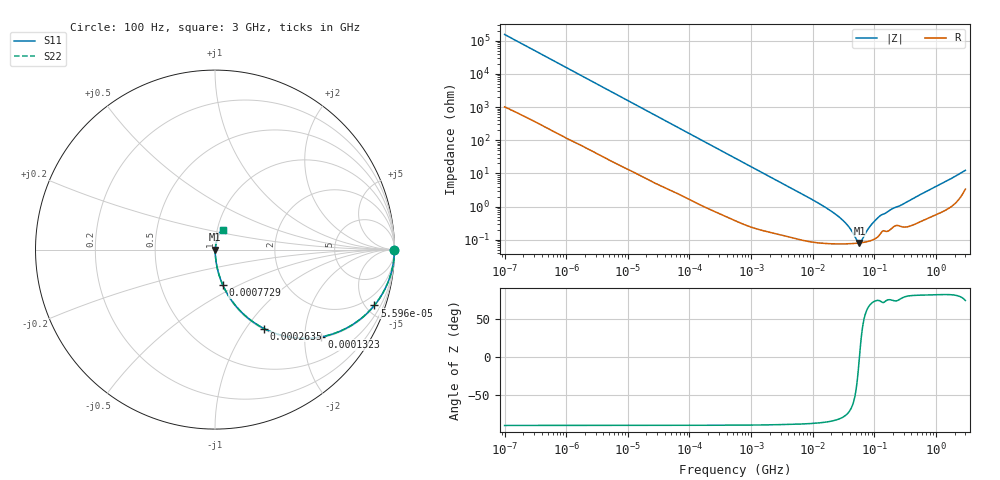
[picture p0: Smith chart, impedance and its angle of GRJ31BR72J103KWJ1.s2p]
!Murata Part Number: GRJ31BR72J103KWJ1
!These Parameters are Measured in Series Mode Connection
!Data Generated on Jun 19, 2026
!  o--ll--o
!Port1  Port2
!  o------o
!Operation Temp=25[degC], DC Bias Voltage=0[V]
!Freq. Start=100[Hz] Stop=3[GHz] 401[Steps]
# Hz S RI R 50
!Freq.(Hz) S11(Real) S11(Imag) S21(Real) S21(Imag) S12(Real) S12(Imag) S22(Real) S22(Imag)
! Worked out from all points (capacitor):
!   401 points, 100 Hz to 3 GHz, reference 50 ohm
!   read as one part in series: C = 10.3 nF near 109 Hz
!   lowest |Z| = 80.8 mohm at 57.2 MHz (marker M1)
!   series resonance near 57.24 MHz, so ESL is about 750 pH
!   S11 on the Smith chart (normalised r, x): 100 Hz: open; 55.95 kHz: 1.06, -5.68; 132.3 kHz: 1.03, -2.42; 263.5 kHz: 1.01, -1.22; 772.9 kHz: 1.01, -0.42; 3 GHz: 1.07, +0.24
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100  1 -0.00065  4.7e-06 0.00065  4.7e-06 0.00065  1 -0.00065
1788  0.9998 -0.0115  0.000221 0.0115  0.000221 0.0115  0.9998 -0.0115
10003  0.9954 -0.0632  0.00455 0.0632  0.00455 0.0632  0.9954 -0.0632
31977  0.9592 -0.1932  0.0408 0.1932  0.0408 0.1932  0.9592 -0.1932
55955  0.8874 -0.3113  0.1126 0.3113  0.1126 0.3113  0.8874 -0.3113
86054  0.7721 -0.4144  0.2279 0.4144  0.2279 0.4144  0.7721 -0.4144
132342  0.5924 -0.4862  0.4076 0.4862  0.4076 0.4862  0.5924 -0.4862
263501  0.273 -0.4398  0.727 0.4398  0.727 0.4398  0.273 -0.4398
547723  0.0828 -0.2692  0.9172 0.2692  0.9172 0.2692  0.0828 -0.2692
772864  0.0445 -0.1993  0.9555 0.1993  0.9555 0.1993  0.0445 -0.1993
2171352  0.00718 -0.0742  0.9928 0.0742  0.9928 0.0742  0.00718 -0.0742
9794414  0.00113 -0.0163  0.9989 0.0163  0.9989 0.0163  0.00113 -0.0163
2.872754e7  0.000774 -0.00431  0.9992 0.00431  0.9992 0.00431  0.000774 -0.00431
3.71925e7  0.000769 -0.00258  0.9992 0.00258  0.9992 0.00258  0.000769 -0.00258
5.248048e7  0.000794 -0.000505  0.9992 0.000505  0.9992 0.000505  0.000794 -0.000505
5.719833e7  0.000808 -4.6e-06  0.9992 4.6e-06  0.9992 4.6e-06  0.000808 -4.6e-06
6.234031e7  0.000825 0.000497  0.9992 -0.000497  0.9992 -0.000497  0.000825 0.000497
8.070971e7  0.000911 0.00205  0.9991 -0.00205  0.9991 -0.00205  0.000911 0.00205
1.000898e8  0.00106 0.00348  0.9989 -0.00348  0.9989 -0.00348  0.00106 0.00348
1.241234e8  0.00152 0.00509  0.9985 -0.00509  0.9985 -0.00509  0.00152 0.00509
1.751444e8  0.00199 0.00738  0.998 -0.00738  0.998 -0.00738  0.00199 0.00738
3e9  0.0456 0.1108  0.9544 -0.1108  0.9544 -0.1108  0.0456 0.1108
